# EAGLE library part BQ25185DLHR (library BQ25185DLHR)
Battery Management NPI 1-CELL 1A STANDALONE LNR HRGR Source: Datasheet
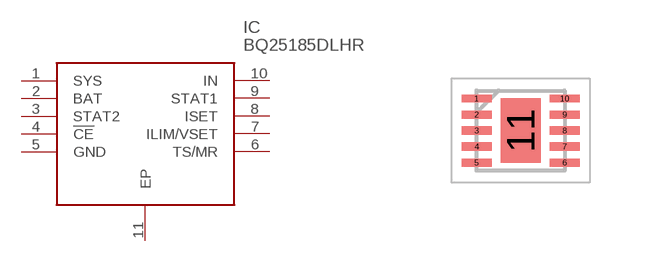
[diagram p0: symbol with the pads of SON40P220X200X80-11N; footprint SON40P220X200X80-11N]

Designator prefix IC

## BQ25185DLHR (Description: Battery Management NPI 1-CELL 1A STANDALONE LNR HRGR; Height: 0.8mm; Manufacturer_Name: Texas Instruments; Manufacturer_Part_Number: BQ25185DLHR; Mouser_Part_Number: 595-BQ25185DLHR; Mouser_Price-Stock: https://www.mouser.co.uk/ProductDetail/Texas-Instruments/BQ25185DLHR?qs=Z%252BL2brAPG1IbO%2FV3RqsaPw%3D%3D)  [SON40P220X200X80-11N]
1  SYS
2  BAT
3  STAT2
4  !CE
5  GND
6  TS/MR
7  ILIM/VSET
8  ISET
9  STAT1
10  IN
11  EP

## Footprint SON40P220X200X80-11N (pad centres in mm)
DLH0010A
smd 0.75 x 0.2: 1 -1.1,0.8; 2 -1.1,0.4; 3 -1.1,0; 4 -1.1,-0.4; 5 -1.1,-0.8; 6 1.1,-0.8; 7 1.1,-0.4; 8 1.1,0; 9 1.1,0.4; 10 1.1,0.8
smd 1 x 1.6: 11 0,0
